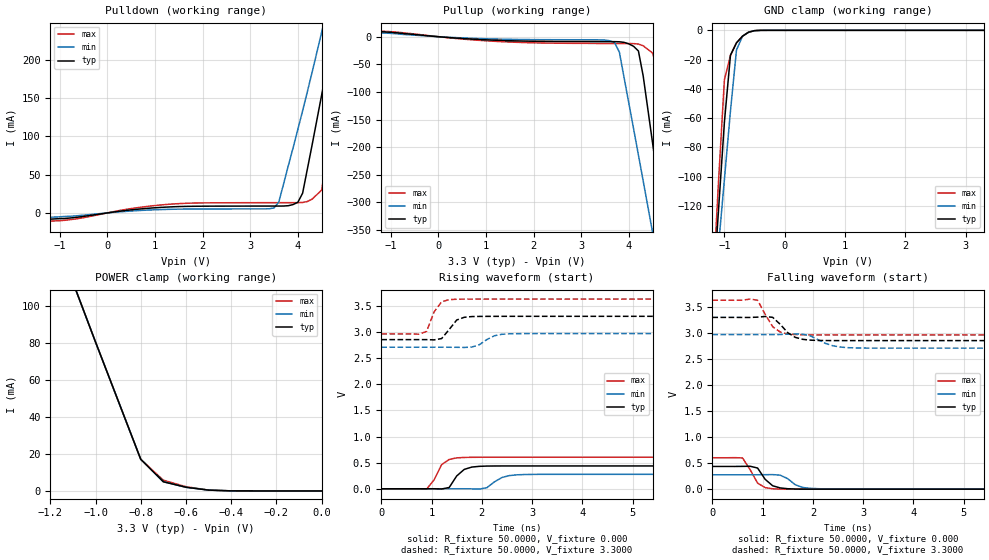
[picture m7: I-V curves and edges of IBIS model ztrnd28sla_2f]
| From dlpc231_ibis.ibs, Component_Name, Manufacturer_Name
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| Model ztrnd28sla_2f
[Model]   ztrnd28sla_2f
Model_type   I/O
Polarity   Non-Inverting
Enable   Active-High
Vinl = 0.8000V
Vinh = 2.0000V
Vmeas = 1.5000V
Cref =50.0000pF
Rref = 0.5000k
Vref =  0.000V
C_comp   0.7000pF   0.7000pF   0.7000pF
[Temperature Range]   25.0000   0.1240k   -40.0000
[Voltage Range]   3.3000V   2.9700V   3.6300V
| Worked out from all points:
|   slope of the pulldown table from 0 to 0.495 V, typ, clamps not added: 125 ohm
|   slope of the pullup table from 0 to 0.495 V, typ, clamps not added: 154 ohm
|   GND clamp passes 1 mA (typ) near -0.57 V on its own axis
|   POWER clamp passes 1 mA (typ) near -0.54 V on its own axis
|   rising waveform, R_fixture 50.0000, V_fixture 0.000: 20-80 % time 232ps typ, 277ps min, 223ps max; typ from 0 V to 0.437 V
|   rising waveform, R_fixture 50.0000, V_fixture 3.3000: 20-80 % time 225ps typ, 271ps min, 202ps max; typ from 2.85 V to 3.3 V
|   falling waveform, R_fixture 50.0000, V_fixture 0.000: 20-80 % time 234ps typ, 279ps min, 219ps max; typ from 0.437 V to 0 V
|   falling waveform, R_fixture 50.0000, V_fixture 3.3000: 20-80 % time 304ps typ, 368ps min, 262ps max; typ from 3.3 V to 2.85 V
[Pulldown]
-3.3V     -12mA      -9mA       -15mA
1.4V      8.055mA    4.828mA    11.75mA
3.5V      8.95mA     6.531mA    13.38mA
3.6V      8.957mA    14.28mA    13.39mA
4V        13.9mA     109.2mA    13.43mA
4.1V      25.79mA    133.7mA    13.62mA
4.2V      57.48mA    158.7mA    14.96mA
4.5V      154.3mA    236.3mA    29.88mA
4.7V      221.6mA    290.9mA    107.1mA
4.9V      291.4mA    348.3mA    191.1mA
5.1V      364.1mA    409.5mA    277.8mA
6.6V      1.038A     961.6mA    1.04A
[Pullup]
-3.3V     7mA        9.3mA      5mA
-1.7V     11.3mA     9.5mA      11.8mA
1.3V      -6.71mA    -4.429mA   -8.856mA
3.7V      -8.962mA   -10.81mA   -12.3mA
3.8V      -9.181mA   -27.96mA   -12.33mA
4.2V      -25.94mA   -214.3mA   -13.34mA
4.3V      -71.03mA   -261.2mA   -16.42mA
4.5V      -194.2mA   -355.7mA   -29.77mA
4.7V      -318.6mA   -450.9mA   -93.02mA
4.9V      -443.8mA   -546.6mA   -249.2mA
5.1V      -569.7mA   -642.7mA   -406.3mA
6.6V      -1.526A    -1.374A    -1.598A
[GND_clamp]
-3.3V     -1.517A    -1.206A    -1.849A
-1.2V     -185.7mA   -194.8mA   -182.8mA
-1.1V     -124mA     -148.1mA   -104.8mA
-1V       -62.54mA   -101.7mA   -33.61mA
-900mV    -17.04mA   -55.16mA   -17.04mA
-800mV    -8.525mA   -13.45mA   -8.525mA
-700mV    -3.999mA   -3.999mA   -3.999mA
-600mV    -1.289mA   -1.289mA   -1.289mA
-500mV    -219.7uA   -252.6uA   -203.6uA
-400mV    -15.61uA   -27.49uA   -11.15uA
3.3V      3.373nA    3.373nA    17.05nA
[POWER_clamp]
-3.3V     1.027A     840.1mA    1.22A
-1.1V     112.7mA    112.7mA    112.7mA
-1V       80.41mA    80.41mA    80.41mA
-800mV    17.08mA    17.08mA    17.08mA
-700mV    4.947mA    4.947mA    5.794mA
-600mV    1.98mA     1.98mA     2.27mA
-500mV    443.8uA    443.8uA    443.8uA
-400mV    34.78uA    34.78uA    34.78uA
0V        3.373nA    3.373nA    57.43nA
[Ramp]
dV/dt_r   0.2620/0.2153n   0.1658/0.2657n   0.3620/0.1932n
dV/dt_f   0.2676/0.2801n   0.1566/0.3580n   0.4002/0.2409n
R_load = 50.0000
[Rising Waveform]
R_fixture = 50.0000
V_fixture = 0.000
V_fixture_min = 0.000
V_fixture_max = 0.000
0s        0V         0V         0V
900ps     122.9uV    -1.063uV   -7.537mV
1.05ns    375uV      -2.46uV    170.8mV
1.2ns     -4.156mV   -2.316uV   462.4mV
1.35ns    24.11mV    37.46uV    561.1mV
1.65ns    370.6mV    269.4uV    599.4mV
2.1ns     434.4mV    20.8mV     603.3mV
2.4ns     436.5mV    215.4mV    603.4mV
2.85ns    436.7mV    272.6mV    603.4mV
14.85ns   436.7mV    276.4mV    603.4mV
[Rising Waveform]
R_fixture = 50.0000
V_fixture = 3.3000
V_fixture_min = 2.9700
V_fixture_max = 3.6300
0s        2.854V     2.709V     2.963V
750ps     2.854V     2.709V     2.958V
900ps     2.854V     2.709V     3.01V
1.05ns    2.849V     2.709V     3.385V
1.2ns     2.874V     2.709V     3.579V
1.5ns     3.229V     2.707V     3.627V
1.8ns     3.295V     2.711V     3.629V
2.25ns    3.299V     2.928V     3.63V
2.7ns     3.3V       2.968V     3.63V
14.85ns   3.3V       2.97V      3.63V
[Falling Waveform]
R_fixture = 50.0000
V_fixture = 0.000
V_fixture_min = 0.000
V_fixture_max = 0.000
0s        436.7mV    276.4mV    603.4mV
600ps     438mV      276.3mV    599.6mV
900ps     405.8mV    276.8mV    116.1mV
1.05ns    189.7mV    278.5mV    30.3mV
1.2ns     65.25mV    280mV      7.281mV
1.35ns    23.78mV    268.7mV    1.584mV
1.65ns    2.623mV    85.04mV    59.12uV
1.8ns     775.1uV    31.72mV    9.641uV
2.25ns    17.95uV    4.779mV    0V
14.85ns   0V         0V         0V
[Falling Waveform]
R_fixture = 50.0000
V_fixture = 3.3000
V_fixture_min = 2.9700
V_fixture_max = 3.6300
0s        3.3V       2.97V      3.63V
900ps     3.305V     2.969V     3.629V
1.2ns     3.301V     2.969V     3.121V
1.35ns    3.167V     2.971V     3.019V
1.5ns     3.006V     2.978V     2.981V
1.65ns    2.916V     2.981V     2.969V
1.95ns    2.863V     2.946V     2.963V
2.4ns     2.854V     2.754V     2.963V
2.85ns    2.854V     2.713V     2.963V
14.85ns   2.854V     2.709V     2.963V
